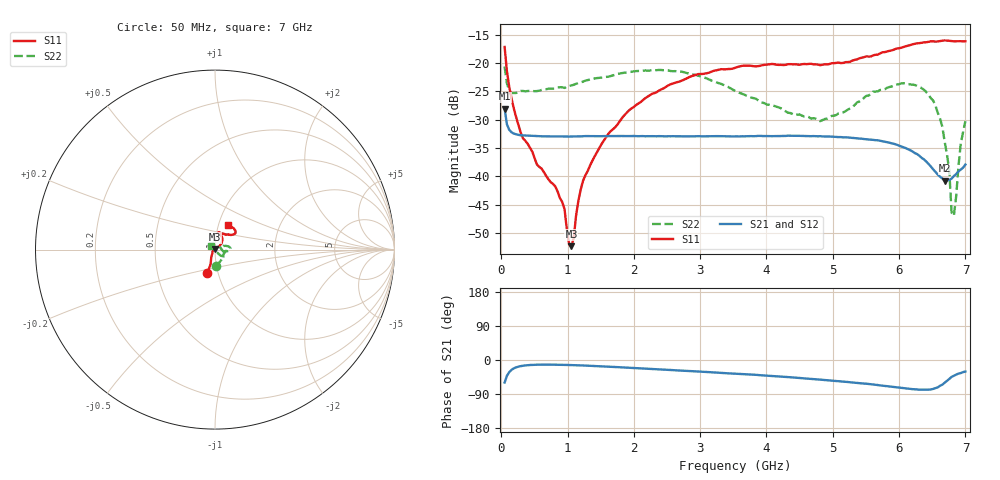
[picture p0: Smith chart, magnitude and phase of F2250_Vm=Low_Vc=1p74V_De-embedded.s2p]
! Integrated Device Technology
! Corporate Headquarters
! 6024 Silver Creek Valley Road
! San Jose, CA 95138  USA
! Phone:  1-408-284-8200
! Toll Free:  1-800-223-1366
! Webpage:  http://www.idt.com/
! Timing and RF Division
! 515 Groton Road, Suite 102
! Westford, MA 01886-6024
! Device:  F2250
! Description: Voltage Variable RF Attenuator
! Frequency:  50.0 -  6000.00 MHz
! Package:  3x3 mm Thin QFN Plastic Package: 16 pin
! Ports:  2 RF, 3 DC
!  Pin  1  = GND
!  Pin  2  = NC
!  Pin  3  = RF1  = Port 1
!  Pin  4  = NC
!  Pin  5  = GND
!  Pin  6  = GND
!  Pin  7  = GND
!  Pin  8  = GND
!  Pin  9  = NC
!  Pin 10  = RF2  = Port 2
!  Pin 11  = NC
!  Pin 12  = GND
!  Pin 13  = GND
!  Pin 14  = VCNTRL
!  Pin 15  = VDD
!  Pin 16  = VMODE
! Vcntrl:  1.740 Volts
! Vmode:  +0.000 Volts
! Vdd:  +3.30  Volts
! Current:  1.187 mA
! Data:  The device was measured on a the F2250 evaluation board which has
!  individual transmission lines to the RF pins.  Data was collected
!  using a calibrated network analyzer.  The evaluation board was
!  de-embedded using a TRL calibration technique.
!  The reference plane is the edge of the package pin.
! Misc:  SN 10
!  Action Tracker AT0258
! Date Measured:  2014-11-26
! Date:  2015-10-15  MJV
! Note:
!  Integrated Device Technology supplies this data as a sample of measured
!  data at the package pin for this product.  Your particular data for this
!  product may vary.
!  Data was taken at 25 degrees C.
!  Integrated Device Technology reserves the right to change this data at anytime.
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# GHz S dB R 50
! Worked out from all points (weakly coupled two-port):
!   201 points, 50 MHz to 7 GHz, reference 50 ohm
!   highest |S21| = -28.07 dB at 50 MHz (marker M1); lowest = -40.8 dB at 6.687 GHz (marker M2)
!   lowest |S11| = -52.4 dB at 1.058 GHz (marker M3), VSWR 1.00, Z = 49.9 + j0.223 ohm
!   |S11| at or under -10 dB: start of sweep to end of sweep
!   |S22| runs from -47.0 to -20.6 dB; largest |S21 - S12| = 9.1e-05
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0.05  -17.16 -108.2  -28.07 -59.4  -28.06 -59.3  -20.62 -86.0
0.1195  -24.19 -111.0  -31.79 -31.9  -31.80 -31.9  -24.86 -39.4
0.29325  -32.30 -126.2  -32.76 -16.1  -32.74 -16.1  -24.93 -16.4
0.84925  -42.69 170.9  -32.96 -12.5  -32.96 -12.5  -24.34 -8.0
0.9535  -45.79 170.6  -32.98 -12.9  -32.97 -12.9  -24.40 -7.9
1.023  -52.08 139.9  -32.99 -13.2  -32.97 -13.2  -24.04 -7.0
1.05775  -52.35 112.3  -32.97 -13.4  -32.97 -13.4  -23.96 -6.6
1.2315  -40.85 40.4  -32.92 -14.4  -32.95 -14.4  -23.29 -7.9
1.61375  -32.53 39.4  -32.91 -17.6  -32.92 -17.6  -22.43 -4.4
2.37825  -24.87 46.7  -32.91 -24.8  -32.92 -24.8  -21.22 3.0
3.525  -20.85 72.2  -32.95 -36.0  -32.96 -36.0  -24.92 21.1
4.7065  -20.22 72.2  -32.90 -50.2  -32.90 -50.2  -29.74 25.1
5.15825  -19.97 57.7  -33.13 -57.2  -33.14 -57.1  -28.72 1.7
5.85325  -17.85 40.3  -34.07 -69.8  -34.09 -69.8  -24.23 -25.9
6.40925  -16.33 41.6  -37.39 -78.5  -37.42 -78.5  -25.11 -41.1
6.54825  -16.21 45.0  -39.22 -74.3  -39.22 -74.3  -27.51 -47.3
6.68725  -16.01 48.7  -40.78 -60.0  -40.79 -59.8  -33.89 -52.9
6.75675  -16.07 51.0  -40.66 -50.0  -40.67 -49.7  -38.93 -62.9
6.7915  -16.12 52.1  -40.42 -44.5  -40.41 -44.3  -46.42 -83.0
6.82625  -16.16 53.4  -39.97 -41.5  -39.98 -41.3  -46.98 -150.7
6.9305  -16.14 59.1  -38.81 -34.5  -38.79 -34.5  -34.25 148.8
7  -16.15 63.1  -37.93 -30.5  -37.90 -30.6  -30.26 142.2
